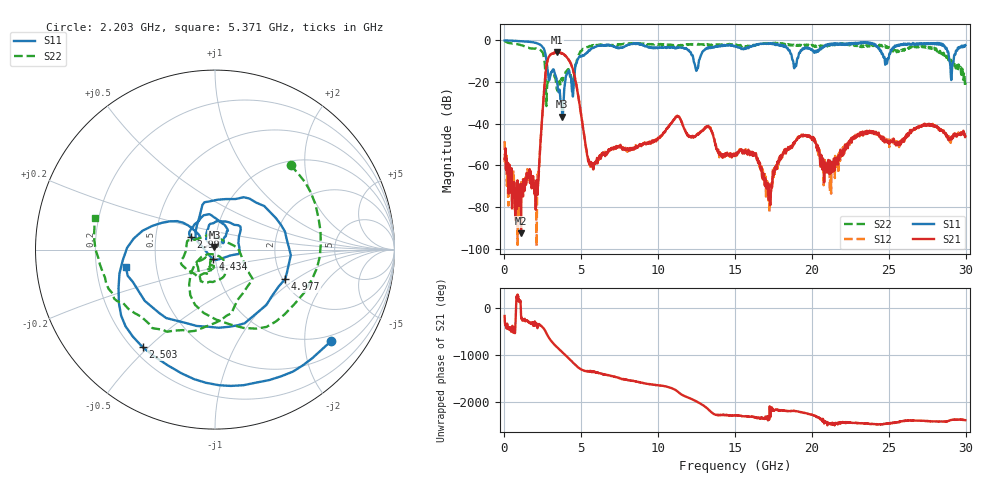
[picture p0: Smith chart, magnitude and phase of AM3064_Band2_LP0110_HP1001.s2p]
# Hz S DB R 50.0
!freq dBS11 angS11 dBS21 angS21 dBS12 angS12 dBS22 angS22
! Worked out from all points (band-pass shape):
!   1600 points, 10 MHz to 29.98 GHz, reference 50 ohm
!   highest |S21| = -5.71 dB at 3.403 GHz (marker M1); lowest = -92.6 dB at 1.078 GHz (marker M2)
!   |S21| within 3 dB of the highest: 2.838 GHz to 4.12 GHz (1.282 GHz wide, 36.9 % of centre)
!   lowest |S11| = -36.6 dB at 3.759 GHz (marker M3), VSWR 1.03, Z = 49.6 + j1.43 ohm
!   |S11| at or under -10 dB: 2.736 GHz to 4.723 GHz (1.987 GHz wide, 53.3 % of centre); 12.31 GHz to 12.65 GHz (334 MHz wide, 2.68 % of centre); 28.95 GHz to 29.21 GHz (257.2 MHz wide, 0.884 % of centre)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
!   |S22| runs from -31.5 to -0.3 dB; largest |S21 - S12| = 0.017
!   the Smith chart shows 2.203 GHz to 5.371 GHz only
!   S11 on the Smith chart (normalised r, x): 2.203 GHz: 0.84, -2.66; 2.503 GHz: 0.24, -0.48; 2.99 GHz: 0.76, +0.11; 4.434 GHz: 0.97, -0.10; 4.977 GHz: 2.06, -0.83; 5.371 GHz: 0.33, -0.09
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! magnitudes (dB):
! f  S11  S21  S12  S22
! 10 MHz  -0.1  -56.9  -48.4  -0.3
! 1.078 GHz  -0.4  -92.6  -78.6  -2.3
! 2.203 GHz  -1.7  -67.7  -65.2  -4.0
! 2.503 GHz  -3.4  -31.7  -31.5  -6.1
! 2.99 GHz  -16.5  -6.9  -6.9  -16.4
! 3.403 GHz  -19.4  -5.7  -5.8  -23.4
! 3.759 GHz  -36.6  -6.3  -6.3  -19.1
! 4.434 GHz  -25.4  -13.5  -13.4  -23.0
! 4.977 GHz  -7.5  -35.1  -35.1  -5.0
! 5.015 GHz  -7.8  -37.1  -36.8  -5.1
! 5.371 GHz  -5.9  -54.9  -53.9  -3.2
! 10 GHz  -3.6  -46.6  -46.4  -1.9
! 11.27 GHz  -3.5  -36.5  -36.2  -2.6
! 15 GHz  -2.7  -55.1  -55.4  -2.0
! 16.3 GHz  -2.1  -55.0  -54.5  -2.2
! 17.16 GHz  -1.6  -68.6  -70.3  -1.5
! 18.25 GHz  -3.2  -52.9  -54.0  -1.9
! 19.99 GHz  -4.4  -46.7  -47.3  -2.2
! 21.1 GHz  -2.3  -62.8  -61.1  -2.4
! 22.97 GHz  -1.5  -44.9  -45.9  -2.3
! 25 GHz  -8.5  -48.6  -47.6  -3.2
! 29.98 GHz  -2.3  -46.0  -46.3  -20.3
